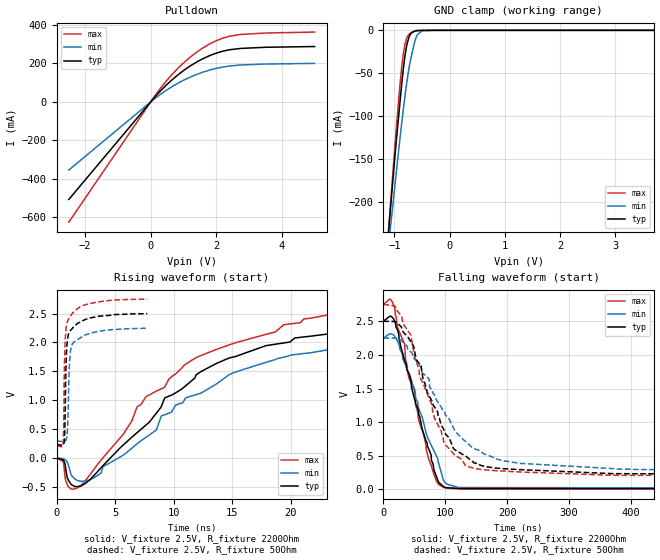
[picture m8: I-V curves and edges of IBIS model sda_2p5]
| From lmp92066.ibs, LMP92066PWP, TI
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|   sda_2p5 Model
[Model]   sda_2p5
Model_type   I/O_open_drain
Polarity   Non-Inverting
Vinl = 0.75
Vinh = 1.75
Vmeas = 1.25
Vref = 2.5
Cref = 100pF
Rref = 2200
|   typ   min   max
|   (nom PVT)   (fast PVT)   (slow PVT)
C_comp   2.070e-12   1.832e-12   2.430e-12
[Model spec]
|subparameter
Vinl   0.75   0.675   0.825
Vinh   1.75   1.575   1.925
| Where nom  PVT is Nominal Process, 2.5V, 25C
|   Fast PVT is Strong Process,  2.75V, -25C
|   Slow PVT is Weak Process,   2.25V, 125C
[Voltage Range]   2.5   2.25   2.75
|Junction Temperature
[Temperature Range]   25   125   -25
[Pullup Reference]   2.5   2.25   2.75
[Pulldown Reference]   0   0   0
[Power Clamp Reference]   2.5   2.25   2.75
[GND Clamp Reference]   0   0   0
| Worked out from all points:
|   slope of the pulldown table from 0 to 0.375 V, typ, clamps not added: 5.3 ohm
|   GND clamp passes 1 mA (typ) near -0.63 V on its own axis
|   falling waveform, V_fixture 2.5V, R_fixture 2200Ohm: 20-80 % time 45.3ns typ, 49.7ns min, 37.8ns max; typ from 2.5 V to 0.006 V
|   rising waveform, V_fixture 2.5V, R_fixture 2200Ohm: 20-80 % time 12.3ns typ, 12.2ns min, 12.6ns max; typ from 0.006 V to 2.49 V
|   falling waveform, V_fixture 2.5V, R_fixture 50Ohm: 20-80 % time 59.2ns typ, 78.5ns min, 52ns max; typ from 2.5 V to 0.234 V
|   rising waveform, V_fixture 2.5V, R_fixture 50Ohm: 20-80 % time 213ps typ, 227ps min, 194ps max; typ from 0.234 V to 2.5 V
[Pulldown]
|   Voltage   I(typ)   I(min)   I(max)
-2.5V     -507.7mA   -354.8mA   -626.2mA
155mV     31.07mA    21.49mA    38.55mA
665.3mV   117.2mA    81.13mA    145.6mA
949.3mV   156.5mA    108.2mA    194.6mA
1.25V     191.9mA    132.5mA    239.2mA
1.55V     221.2mA    152.4mA    276.4mA
1.849V    244.5mA    168.1mA    306.4mA
2.148V    261.6mA    179.8mA    328.9mA
2.448V    272.5mA    187.6mA    343.3mA
2.752V    278.5mA    192.2mA    351.2mA
3.492V    284.3mA    197.1mA    358.6mA
5V        288.3mA    200.5mA    363.5mA
[GND Clamp]
|   Voltage   I(typ)   I(min)   I(max)
-2.5V     -1.253A    -1.02A     -1.321A
-1.31V    -391.2mA   -373.1mA   -405.3mA
-1.02V    -168.5mA   -198.7mA   -159mA
-913.3mV  -93.43mA   -134.1mA   -73.33mA
-866.5mV  -61.58mA   -107.3mA   -41.74mA
-837.5mV  -44.09mA   -91.43mA   -26.68mA
-806mV    -28.33mA   -75.09mA   -15.29mA
-772.5mV  -16.03mA   -59.13mA   -8.28mA
-695mV    -3.257mA   -30.53mA   -2.512mA
-597mV    -426.7uA   -6.633mA   -405.1uA
-497.5mV  -38.44uA   -605.2uA   -28uA
5V        0A         0A         0A
[POWER Clamp]
|   Voltage   I(typ)   I(min)   I(max)
-2.5V     0A         0A         0A
0V        0A         0A         0A
5V        0A         0A         0A
[Ramp]
R_load = 2200
|   typ   min   max
dV/dt_r   1.49667/1.24836e-08   1.34597/1.24945e-08   1.64704/1.266e-08
dV/dt_f   1.49662/4.49951e-08   1.34593/4.97567e-08   1.64699/3.77634e-08
[Falling Waveform]
V_fixture = 2.5V
V_fixture_min = 2.25V
V_fixture_max = 2.75V
R_fixture = 2200Ohm
|   Time   V(typ)   V(min)   V(max)
0s        2.5V       2.25V      2.75V
11.82ns   2.575V     2.314V     2.823V
19.92ns   2.463V     2.247V     2.578V
34.12ns   1.917V     1.892V     2.164V
39.92ns   1.741V     1.758V     1.706V
50.4ns    1.339V     1.493V     1.469V
72.95ns   607.4mV    743.7mV    457.2mV
89.15ns   107.2mV    392.2mV    75.29mV
100ns     30.16mV    98mV       22.05mV
1.57us    5.55mV     7.208mV    4.932mV
[Rising Waveform]
V_fixture = 2.5V
V_fixture_min = 2.25V
V_fixture_max = 2.75V
R_fixture = 2200Ohm
|   Time   V(typ)   V(min)   V(max)
0s        5.55mV     7.208mV    4.931mV
548.4ps   -25.03mV   -3.251mV   -48.18mV
994ps     -369.6mV   -104mV     -484.8mV
1.772ns   -487.8mV   -380.5mV   -510.2mV
6.886ns   445.8mV    253mV      893mV
10.89ns   1.229V     996.2mV    1.606V
14.75ns   1.734V     1.446V     1.96V
21.12ns   2.096V     1.81V      2.408V
31.2ns    2.373V     2.102V     2.588V
56.36ns   2.492V     2.241V     2.746V
[Falling Waveform]
V_fixture = 2.5V
V_fixture_min = 2.25V
V_fixture_max = 2.75V
R_fixture = 50Ohm
|   Time   V(typ)   V(min)   V(max)
0s        2.5V       2.25V      2.75V
18.5ns    2.497V     2.25V      2.729V
44.11ns   2.199V     2.048V     2.3V
48.95ns   2.127V     1.95V      2.05V
70.8ns    1.445V     1.669V     1.421V
98.55ns   871.4mV    1.158V     686mV
113.2ns   607.6mV    913.5mV    532.2mV
132.5ns   500.1mV    716.1mV    355.4mV
218.4ns   296.2mV    391.2mV    261.5mV
448.6ns   233.8mV    296mV      210.3mV
[Rising Waveform]
V_fixture = 2.5V
V_fixture_min = 2.25V
V_fixture_max = 2.75V
R_fixture = 50Ohm
|   Time   V(typ)   V(min)   V(max)
0s        233.8mV    295.2mV    210.3mV
577.4ps   233.4mV    289.9mV    293.8mV
681.6ps   329.9mV    295.8mV    1.661V
730.2ps   694.2mV    299.7mV    2.026V
776.9ps   1.329V     306.9mV    2.143V
860.9ps   1.863V     346.8mV    2.313V
962ps     2.078V     608.1mV    2.376V
1.182ns   2.208V     1.823V     2.457V
2.549ns   2.404V     2.138V     2.657V
7.75ns    2.499V     2.248V     2.749V
